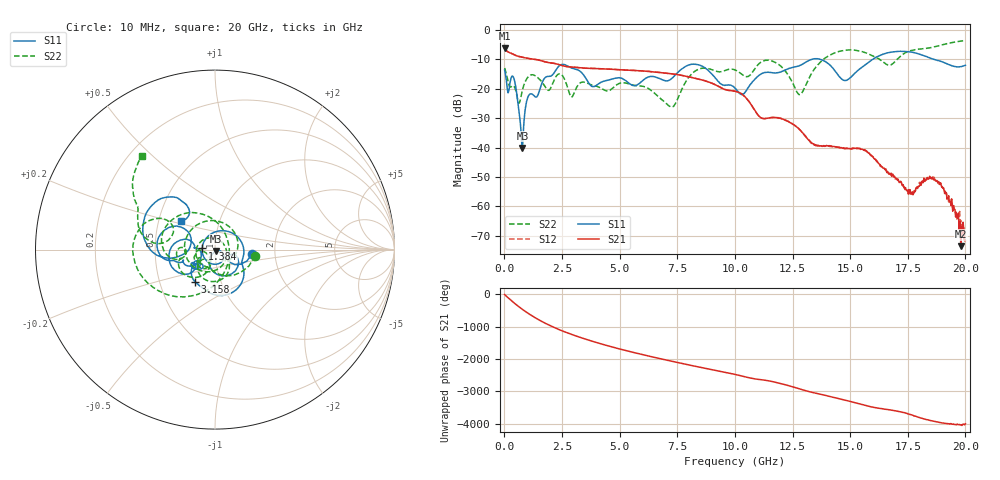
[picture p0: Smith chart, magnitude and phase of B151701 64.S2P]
!  2-Port S-parameters saved by WinCal
! VAR MeasName=S-Parameters (CALIBRATED_DATA) read from VNA (N5244A)
! VAR MeasDate=2015-12-24 19:17:32
! VAR NAME=B151701 64
! VAR FILENAME=B151701 64.S2P
! VAR DATE=2015-12-24 19:17:32
! VAR PHYS_PORTS=1,3
# Hz S DB R 50
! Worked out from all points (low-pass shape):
!   801 points, 10 MHz to 20 GHz, reference 50 ohm
!   highest |S21| = -6.29 dB at 10 MHz (marker M1); lowest = -73.5 dB at 19.8 GHz (marker M2)
!   |S21| within 3 dB of the highest: start of sweep to 787.8 MHz
!   lowest |S11| = -40.1 dB at 784.6 MHz (marker M3), VSWR 1.02, Z = 50.6 - j0.755 ohm
!   |S11| at or under -10 dB: start of sweep to 13.34 GHz; 13.7 GHz to 15.98 GHz (2.276 GHz wide, 15.3 % of centre); 18.64 GHz to end of sweep
!   |S22| runs from -26.3 to -3.6 dB; largest |S21 - S12| = 0.0012
!   S11 on the Smith chart (normalised r, x): 10 MHz: 1.52, -0.07; 1.384 GHz: 0.87, +0.01; 3.158 GHz: 0.75, -0.28; 20 GHz: 0.65, +0.22
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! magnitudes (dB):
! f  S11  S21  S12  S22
! 10 MHz  -13.6  -6.3  -6.3  -12.9
! 434.8 MHz  -17.1  -8.5  -8.5  -19.4
! 784.6 MHz  -40.1  -9.3  -9.3  -20.4
! 1.034 GHz  -22.6  -9.7  -9.7  -16.0
! 1.384 GHz  -22.8  -10.1  -10.1  -15.8
! 1.909 GHz  -15.8  -11.1  -11.1  -20.5
! 2.409 GHz  -12.0  -11.9  -11.9  -15.0
! 3.158 GHz  -13.5  -12.8  -12.8  -19.2
! 3.358 GHz  -14.6  -12.9  -12.9  -17.8
! 6.682 GHz  -16.4  -14.4  -14.4  -22.7
! 7.306 GHz  -16.2  -15.0  -15.0  -26.1
! 8.306 GHz  -11.7  -16.5  -16.5  -13.8
! 10.01 GHz  -19.8  -20.9  -20.8  -13.6
! 11.63 GHz  -14.6  -29.8  -29.7  -10.6
! 12.8 GHz  -12.1  -33.8  -33.9  -22.0
! 13.35 GHz  -10.0  -38.6  -38.5  -14.4
! 14.8 GHz  -17.2  -40.3  -40.2  -6.9
! 16.68 GHz  -7.7  -49.0  -48.3  -12.0
! 17.6 GHz  -7.5  -54.3  -55.5  -7.1
! 18.85 GHz  -10.5  -51.7  -52.4  -5.4
! 19.8 GHz  -12.5  -73.5  -64.8  -3.8
! 20 GHz  -12.0  -71.6  -69.1  -3.6
